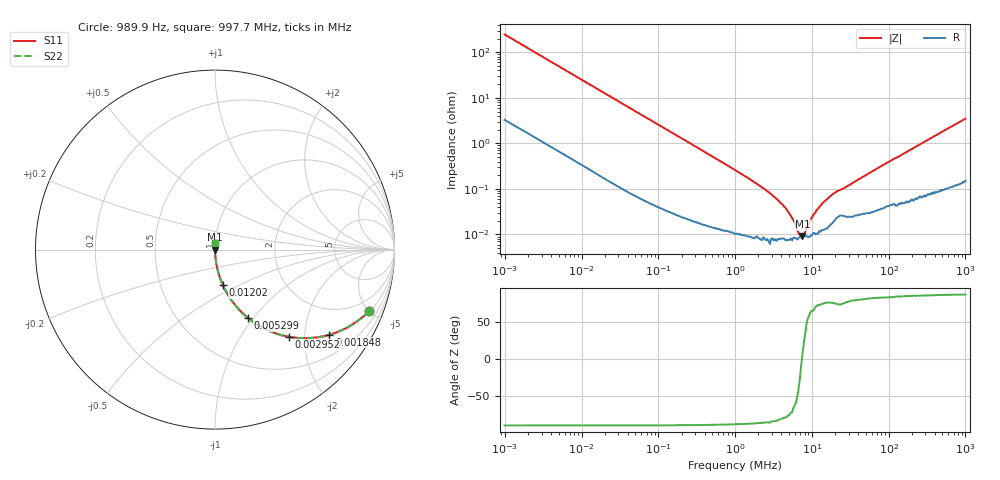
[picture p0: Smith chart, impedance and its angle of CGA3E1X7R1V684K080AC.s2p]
! S-Parameter Data Generated by TDK Corporation
! Copyright(C) 2022 TDK Corporation.
! All Rights Reserved.
! TDK P/N: CGA3E1X7R1V684K080AC (Multilayer Ceramic Chip Capacitor)
! Property: C=680nF
! Size(LxWxT): 1.6x0.8x0.8mm
! Model Type: s2p (Touchstone File Format Version 1.0)
! Frequency: DC=Yes Start=0.00098985MHz Stop=997.74MHz 408points Log-sweep
! Model Generated on Apr. 15, 2022
! Port Assignments:
!  1 ---| |--- 2
! Applicable Conditions:
!  Temperature = 25 degC
!  DC Bias Voltage = 0 V
!  Small Signal Operation
! Terms and conditions regarding TDK Simulation Models
! (1)This simulation model is being provided solely for informational purposes. Please refer to the specifications of the products in terms of detailed characteristics of such products.
! (2)In no event shall TDK Corporation of any of its subsidiaries be liable for any loss or damage arising, directly or indirectly,
!  From any information contained in this simulation model, including, but not limited to loss or damages arising from any inaccuracies, omissions or errors in connection with such information.
! (3)Any and all copyrights on this simulation model are owned by TDK Corporation.
!  Duplication or redistribution of this simulation model without prior written permission from TDK Corporation is prohibited.
! (4)This simulation model is subject to any modification or change without any prior notice.
! (5)Neither TDK Corporation nor any of its subsidiaries shall make any warranty, express or implied,
!  Including but not limited to the correctness, implied warranties of merchantability and fitness for a particular purpose with respect to this simulation models.
! (6)The use of this simulation model shall be deemed to have consented to the terms and conditions hereof.
# Hz S MA R 50
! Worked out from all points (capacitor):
!   407 points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, 989.9 Hz to 997.7 MHz, reference 50 ohm
!   read as one part in series: C = 649 nF near 1.07 kHz
!   lowest |Z| = 9 mohm at 7.517 MHz (marker M1)
!   series resonance near 7.396 MHz, so ESL is about 710 pH
!   S11 on the Smith chart (normalised r, x): 989.9 Hz: 1.07, -4.95; 1.848 kHz: 1.04, -2.66; 2.951 kHz: 1.02, -1.67; 5.299 kHz: 1.01, -0.94; 12.03 kHz: 1.01, -0.42; 997.7 MHz: 1.00, +0.07
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989.85  0.9229 -21.9  0.3731 67.3  0.3731 67.3  0.9229 -21.9
1848  0.7944 -36.6  0.5968 52.6  0.5968 52.6  0.7944 -36.6
2951.5  0.6373 -49.6  0.762 39.6  0.762 39.6  0.6373 -49.6
5299.3  0.4219 -64.3  0.9009 25.0  0.9009 25.0  0.4219 -64.3
10287  0.2355 -75.6  0.9687 13.6  0.9687 13.6  0.2355 -75.6
12025  0.2036 -77.5  0.9763 11.7  0.9763 11.7  0.2036 -77.5
30673  0.08247 -84.5  0.9955 4.7  0.9955 4.7  0.08247 -84.5
102820  0.02502 -87.7  0.9993 1.4  0.9993 1.4  0.02502 -87.7
1027600  0.002516 -87.5  0.9999 0.1  0.9999 0.1  0.002516 -87.5
2242600  0.001076 -85.9  0.9999 0.1  0.9999 0.1  0.001076 -85.9
3581800  0.0005698 -82.0  0.9999 0.0  0.9999 0.0  0.0005698 -82.0
4894000  0.0003148 -76.2  0.9999 0.0  0.9999 0.0  0.0003148 -76.2
5720600  0.0002063 -65.8  0.9999 0.0  0.9999 0.0  0.0002063 -65.8
6686900  0.0001088 -40.1  0.9999 0.0  0.9999 0.0  0.0001088 -40.1
6952900  9.713e-05 -26.7  0.9999 0.0  0.9999 0.0  9.713e-05 -26.7
7517300  9.003e-05 6.3  0.9999 -0.0  0.9999 -0.0  9.003e-05 6.3
8450800  0.0001345 46.6  0.9999 -0.0  0.9999 -0.0  0.0001345 46.6
1.0271e7  0.000254 65.5  0.9999 -0.0  0.9999 -0.0  0.000254 65.5
1.3497e7  0.0004753 74.8  0.9999 -0.0  0.9999 -0.0  0.0004753 74.8
1.9176e7  0.0007999 75.9  0.9998 -0.0  0.9998 -0.0  0.0007999 75.9
1.0266e8  0.004038 83.6  0.9996 -0.2  0.9996 -0.2  0.004038 83.6
9.9774e8  0.03481 85.5  0.9979 -2.0  0.9979 -2.0  0.03481 85.5
